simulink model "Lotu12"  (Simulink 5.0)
settings: Solver=ode45  StartTime=0.0  StopTime=10.0  RelTol=1e-3

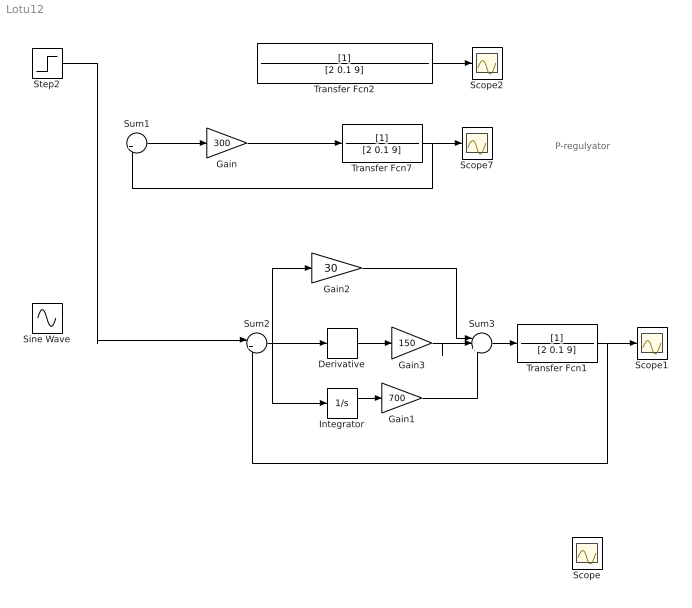
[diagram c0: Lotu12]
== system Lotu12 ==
  note: P-regulyator
  Derivative : Derivative
  Gain : Gain  Gain=300
  Gain1 : Gain  Gain=700
  Gain2 : Gain  Gain=30
  Gain3 : Gain  Gain=150
  Integrator : Integrator
  Scope{,1..2,7} (4 alike) : Scope
  Sine Wave : Sin  SampleTime=0
  Step2 : Step  Time=0  SampleTime=0
  Sum1 : Sum  Inputs=|+-
  Sum2 : Sum  Inputs=|+-
  Sum3 : Sum  Inputs=|+++
  Transfer Fcn1 : TransferFcn  Denominator=[2 0.1 9]
  Transfer Fcn2 : TransferFcn  Denominator=[2 0.1 9]
  Transfer Fcn7 : TransferFcn  Denominator=[2 0.1 9]
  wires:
  Step2/1 -> Sum2/1
  Transfer Fcn2/1 -> Scope2/1
  Transfer Fcn7/1 -> Scope7/1, Sum1/2
  Gain/1 -> Transfer Fcn7/1
  Sum1/1 -> Gain/1
  Transfer Fcn1/1 -> Scope1/1, Sum2/2
  Sum2/1 -> Gain2/1, Derivative/1, Integrator/1
  Sum3/1 -> Transfer Fcn1/1
  Gain2/1 -> Sum3/1
  Integrator/1 -> Gain1/1
  Derivative/1 -> Gain3/1
  Gain3/1 -> Sum3/2
  Gain1/1 -> Sum3/3
